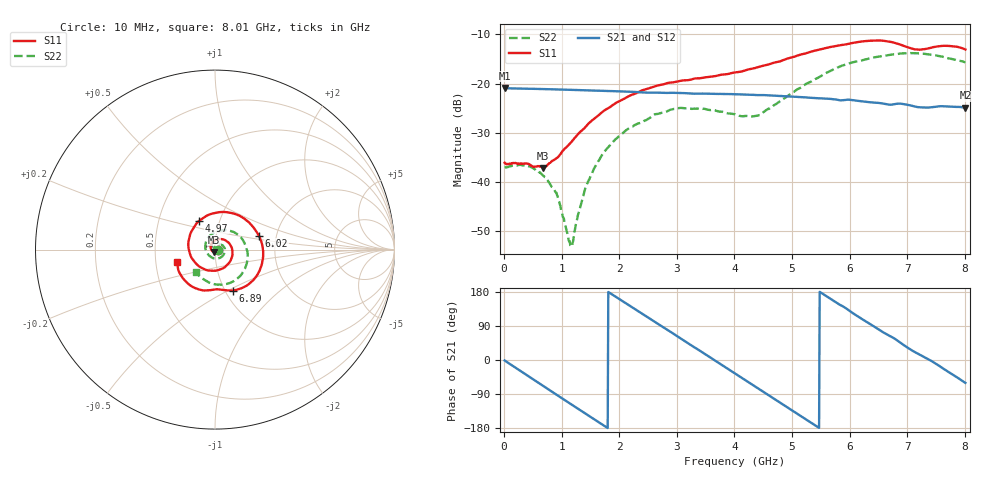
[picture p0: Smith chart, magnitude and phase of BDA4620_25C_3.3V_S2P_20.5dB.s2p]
!Agilent Technologies,E5071B,MY42404982,A.09.10
!Date: Wed May 06 08:53:10 2026
!Data & Calibration Information:
!Freq	S11:SOLT2(ON)	S21:SOLT2(ON)	S12:SOLT2(ON)	S22:SOLT2(ON)
# Hz S RI R 50
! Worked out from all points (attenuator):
!   801 points, 10 MHz to 8.01 GHz, reference 50 ohm
!   highest |S21| = -20.90 dB at 10 MHz (marker M1); lowest = -24.9 dB at 8.01 GHz (marker M2)
!   lowest |S11| = -37.1 dB at 680 MHz (marker M3), VSWR 1.03, Z = 49.6 - j1.34 ohm
!   |S11| at or under -10 dB: start of sweep to end of sweep
!   |S22| runs from -53.0 to -13.8 dB; largest |S21 - S12| = 0.00037
!   S11 on the Smith chart (normalised r, x): 10 MHz: 1.03, -0.00; 4.97 GHz: 0.80, +0.27; 6.02 GHz: 1.62, +0.26; 6.89 GHz: 1.08, -0.53; 8.01 GHz: 0.65, -0.10
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1e7  0.0157 -0.00107  0.0901 -0.0019  0.0902 -0.00193  0.014 -0.000487
4.3e8  0.00808 -0.013  0.0643 -0.0611  0.0644 -0.0613  0.0135 -0.00521
6.8e8  -0.00361 -0.0135  0.0323 -0.082  0.0322 -0.082  0.00924 -0.00713
9.2e8  -0.0162 -0.00686  -0.00379 -0.0872  -0.00388 -0.0873  0.00353 -0.0065
1.16e9  -0.0236 0.00868  -0.0384 -0.0775  -0.0386 -0.0776  -0.00194 -0.00113
1.35e9  -0.0233 0.024  -0.0609 -0.0605  -0.061 -0.0605  -0.00413 0.00481
1.53e9  -0.0164 0.0391  -0.0759 -0.0387  -0.076 -0.0387  -0.00382 0.0117
1.77e9  0.00275 0.0545  -0.0841 -0.00499  -0.0842 -0.00503  0.00052 0.0213
2.14e9  0.0464 0.0566  -0.0695 0.0453  -0.0696 0.0453  0.017 0.0298
2.68e9  0.096 0.000373  -0.00645 0.0806  -0.00641 0.0808  0.0454 0.0195
3.47e9  0.0213 -0.1132  0.0755 0.0238  0.0757 0.0238  0.0408 -0.0377
4.01e9  -0.0955 -0.0879  0.0634 -0.0454  0.0635 -0.0455  -0.0116 -0.0475
4.42e9  -0.1475 0.00915  0.0187 -0.0742  0.0186 -0.0743  -0.046 -0.0127
4.97e9  -0.0872 0.1611  -0.0479 -0.0564  -0.048 -0.0565  -0.0354 0.0698
5.35e9  0.0362 0.2096  -0.0699 -0.0154  -0.07 -0.0155  0.0232 0.1038
6.02e9  0.2451 0.0755  -0.0416 0.0544  -0.0417 0.0544  0.152 0.0585
6.35e9  0.2639 -0.0683  -0.00597 0.0644  -0.00605 0.0645  0.1801 -0.0113
6.68e9  0.1814 -0.1977  0.0262 0.0553  0.0263 0.0554  0.1717 -0.0925
6.89e9  0.0978 -0.2281  0.0444 0.044  0.0445 0.0442  0.1467 -0.1397
7.19e9  0.0142 -0.2209  0.0554 0.0161  0.0555 0.0162  0.0795 -0.1873
7.56e9  -0.0979 -0.2188  0.0566 -0.0161  0.0568 -0.016  -0.0158 -0.1897
8.01e9  -0.2105 -0.0714  0.0281 -0.0495  0.0282 -0.0496  -0.1044 -0.1267
